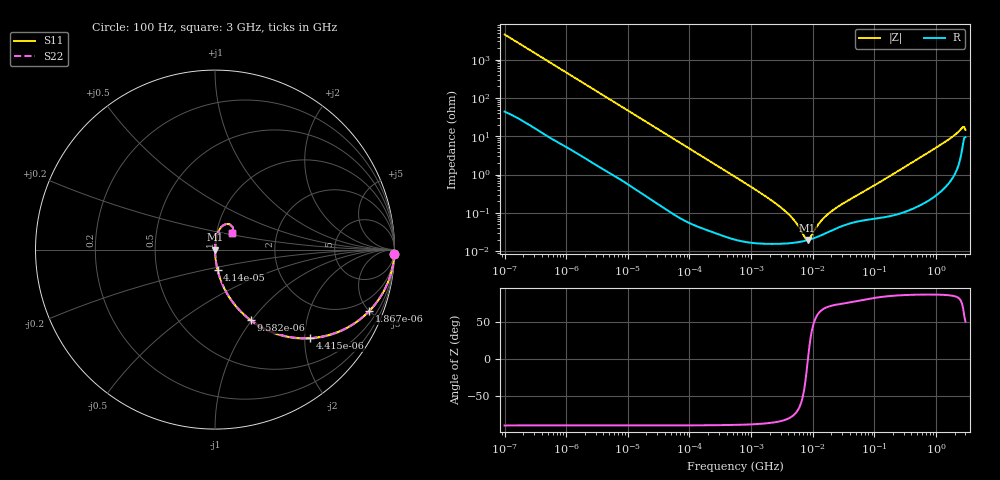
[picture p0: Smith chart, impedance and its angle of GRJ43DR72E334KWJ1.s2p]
!Murata Part Number: GRJ43DR72E334KWJ1
!These Parameters are Measured in Series Mode Connection
!Data Generated on Jun 19, 2026
!  o--ll--o
!Port1  Port2
!  o------o
!Operation Temp=25[degC], DC Bias Voltage=0[V]
!Freq. Start=100[Hz] Stop=3[GHz] 401[Steps]
# Hz S RI R 50
!Freq.(Hz) S11(Real) S11(Imag) S21(Real) S21(Imag) S12(Real) S12(Imag) S22(Real) S22(Imag)
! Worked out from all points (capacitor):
!   401 points, 100 Hz to 3 GHz, reference 50 ohm
!   read as one part in series: C = 348 nF near 109 Hz
!   lowest |Z| = 19.5 mohm at 8.245 MHz (marker M1)
!   series resonance near 8.359 MHz, so ESL is about 1 nH
!   S11 on the Smith chart (normalised r, x): 100 Hz: 2, -91; 1.867 kHz: 1.06, -4.99; 4.415 kHz: 1.02, -2.12; 9.582 kHz: 1.01, -0.98; 41.4 kHz: 1.00, -0.23; 3 GHz: 1.19, +0.23
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100  0.9993 -0.0219  0.000692 0.0219  0.000692 0.0219  0.9993 -0.0219
536  0.9855 -0.1142  0.0145 0.1142  0.0145 0.1142  0.9855 -0.1142
1788  0.8687 -0.332  0.1313 0.332  0.1313 0.332  0.8687 -0.332
1867  0.8588 -0.3425  0.1412 0.3425  0.1412 0.3425  0.8588 -0.3425
4415  0.5296 -0.4933  0.4704 0.4933  0.4704 0.4933  0.5296 -0.4933
9582  0.198 -0.3926  0.802 0.3926  0.802 0.3926  0.198 -0.3926
16060  0.0826 -0.2696  0.9174 0.2696  0.9174 0.2696  0.0826 -0.2696
31977  0.0232 -0.1451  0.9768 0.1451  0.9768 0.1451  0.0232 -0.1451
41399  0.0143 -0.1133  0.9857 0.1133  0.9857 0.1133  0.0143 -0.1133
116311  0.00218 -0.0411  0.9978 0.0411  0.9978 0.0411  0.00218 -0.0411
547723  0.000276 -0.00878  0.9997 0.00878  0.9997 0.00878  0.000276 -0.00878
3339322  0.000159 -0.00121  0.9998 0.00121  0.9998 0.00121  0.000159 -0.00121
4919190  0.000166 -0.000638  0.9998 0.000638  0.9998 0.000638  0.000166 -0.000638
7565221  0.000187 -0.000113  0.9998 0.000113  0.9998 0.000113  0.000187 -0.000113
8245314  0.000194 -1.53e-05  0.9998 1.53e-05  0.9998 1.53e-05  0.000194 -1.53e-05
9794414  0.000211 0.000179  0.9998 -0.000179  0.9998 -0.000179  0.000211 0.000179
1.323817e7  0.000254 0.000524  0.9997 -0.000524  0.9997 -0.000524  0.000254 0.000524
2.035898e7  0.000348 0.00106  0.9997 -0.00106  0.9997 -0.00106  0.000348 0.00106
1.751444e8  0.000894 0.00894  0.9991 -0.00894  0.9991 -0.00894  0.000894 0.00894
1.324213e9  0.00861 0.0664  0.9914 -0.0664  0.9914 -0.0664  0.00861 0.0664
2.636591e9  0.0626 0.1426  0.9374 -0.1426  0.9374 -0.1426  0.0626 0.1426
3e9  0.0965 0.094  0.9035 -0.094  0.9035 -0.094  0.0965 0.094
